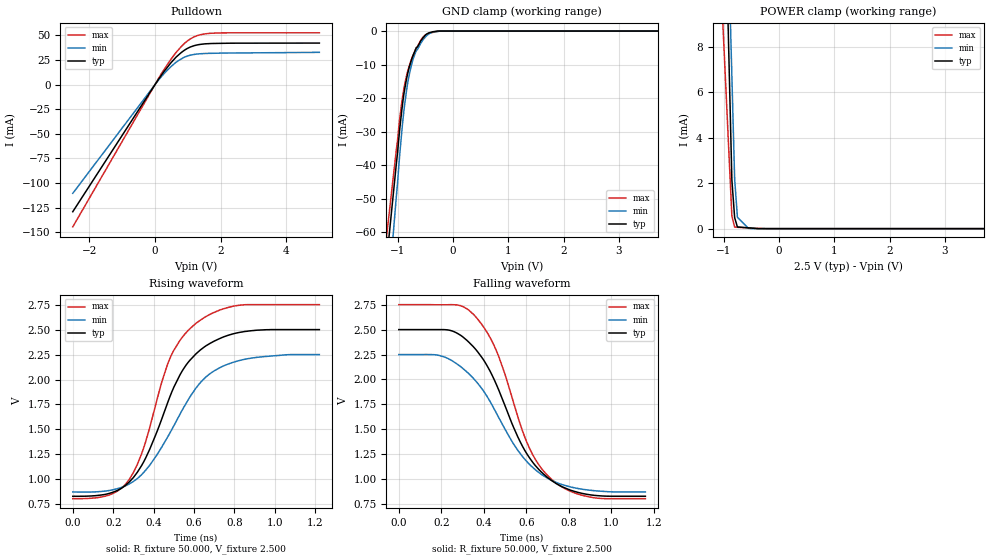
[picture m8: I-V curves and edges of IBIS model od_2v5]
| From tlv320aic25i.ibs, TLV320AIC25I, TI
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[Model]   od_2v5
Model_type I/O_open_drain
Vinl=7.500E-01
Vinh=1.750E+00
Vref=2.500E+00
Rref=5.000E+02
Cref=2.000E-11
Vmeas=1.250E+00
C_comp   1.070E-12   1.070E-12   1.070E-12
[Voltage Range]   2.500E+00   2.250E+00   2.750E+00
[POWER Clamp Reference]   2.500E+00   2.250E+00   2.750E+00
[GND Clamp Reference]   0.000E+00   0.000E+00   0.000E+00
[Pullup Reference]   2.500E+00   2.250E+00   2.750E+00
[Pulldown Reference]   0.000E+00   0.000E+00   0.000E+00
[Temperature Range]   25   85   -40
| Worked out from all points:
|   slope of the pulldown table from 0 to 0.375 V, typ, clamps not added: 21.4 ohm
|   GND clamp passes 1 mA (typ) near -0.48 V on its own axis
|   POWER clamp passes 1 mA (typ) near -0.82 V on its own axis
|   rising waveform, R_fixture 50.000, V_fixture 2.500: 20-80 % time 221ps typ, 251ps min, 192ps max; typ from 0.83 V to 2.5 V
|   falling waveform, R_fixture 50.000, V_fixture 2.500: 20-80 % time 225ps typ, 249ps min, 200ps max; typ from 2.5 V to 0.83 V
[GND Clamp]
-2.5V     -282.2mA   -343.8mA   -252mA
-1.02V    -39.29mA   -48.97mA   -35.15mA
-960mV    -29.11mA   -36.7mA    -26.01mA
-900mV    -20.5mA    -26mA      -18.6mA
-840mV    -14.43mA   -18.03mA   -13.54mA
-800mV    -11.46mA   -13.99mA   -11.01mA
-720mV    -7.326mA   -8.411mA   -7.221mA
-660mV    -4.968mA   -5.824mA   -4.891mA
-540mV    -2.01mA    -2.589mA   -1.8mA
-440mV    -589.5uA   -910.3uA   -693.6uA
-220mV    0A         0A         0A
5V        0A         0A         0A
[POWER Clamp]
-2.5V     167.8mA    155.3mA    86.3mA
-1.05V    22.23mA    24.71mA    10.95mA
-850mV    2.14mA     6.693mA    557.3uA
-800mV    484.1uA    2.189mA    65.39uA
-750mV    73.7uA     504.3uA    59.17uA
-550mV    34.39uA    10.79uA    34.25uA
-375mV    0A         0A         12.46uA
5V        0A         0A         0A
[Pulldown]
-2.5V     -129.2mA   -110.5mA   -144.6mA
200mV     9.967mA    8.366mA    11.43mA
460mV     21.18mA    17.48mA    24.6mA
640mV     27.95mA    22.74mA    32.71mA
820mV     33.17mA    26.55mA    39.41mA
1V        37.1mA     29.26mA    44.8mA
1.26V     40.22mA    31.06mA    49.57mA
1.68V     41.79mA    31.85mA    52.24mA
5V        42.29mA    32.85mA    52.7mA
[Rising Waveform]
R_fixture = 50.000
V_fixture = 2.500
V_fixture_min = 2.250
V_fixture_max = 2.750
|  time   V(typ)   V(min)   V(max)
0s        829.9mV    873.1mV    805.7mV
180ps     858.4mV    887.7mV    842.4mV
280ps     974.3mV    954.2mV    1V
350ps     1.172V     1.067V     1.31V
480ps     1.825V     1.462V     2.209V
540ps     2.081V     1.689V     2.419V
610ps     2.258V     1.916V     2.564V
700ps     2.385V     2.087V     2.673V
820ps     2.47V      2.188V     2.743V
1.22ns    2.5V       2.25V      2.75V
[Falling Waveform]
R_fixture = 50.000
V_fixture = 2.500
V_fixture_min = 2.250
V_fixture_max = 2.750
|  time   V(typ)   V(min)   V(max)
0s        2.5V       2.25V      2.75V
210ps     2.5V       2.229V     2.749V
290ps     2.444V     2.13V      2.74V
360ps     2.306V     1.99V      2.633V
460ps     1.945V     1.659V     2.283V
560ps     1.424V     1.289V     1.626V
620ps     1.199V     1.138V     1.288V
740ps     957.5mV    968.8mV    962.3mV
910ps     841.2mV    887.5mV    817.9mV
1.16ns    829.9mV    873.1mV    805.7mV
[Ramp]
dV/dt_r   1.002E+00/2.208E-10   8.261E-01/2.502E-10   1.167E+00/1.911E-10
dV/dt_f   1.002E+00/2.247E-10   8.261E-01/2.490E-10   1.167E+00/2.002E-10
R_load = 50
